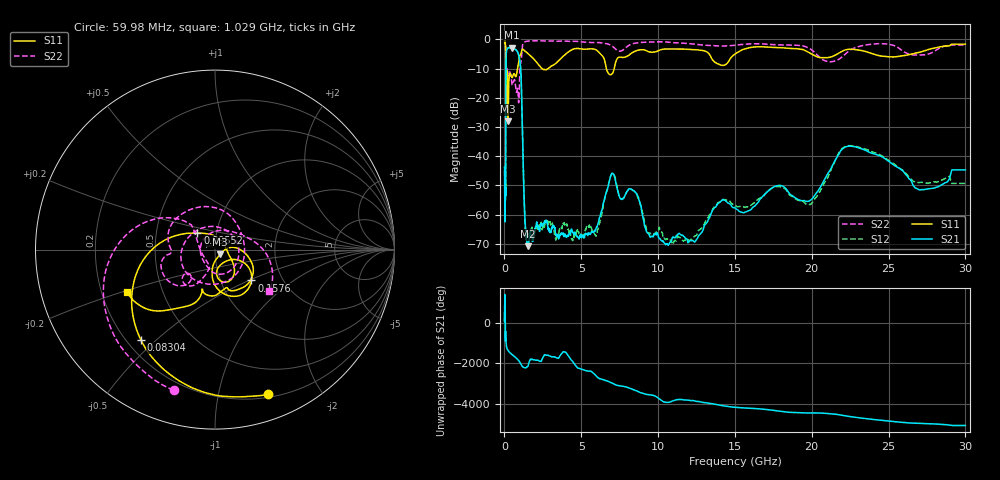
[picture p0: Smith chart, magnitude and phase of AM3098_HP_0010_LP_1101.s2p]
! Date/Time: Thu, Feb 28, 2019 8:33 AM
! Network Analyzer: Agilent Technologies E8364B Rev: A.07.50.67
! Sweep from 0.010 to 30.000 GHz, 1601 Points, Sweep Type: LOG
! Power Supply: 5.022 V, 0.002 A
# Hz S DB R 50
!freq MagS11 AngS11 MagS21 AngS21 MagS12 AngS12 MagS22 AngS22
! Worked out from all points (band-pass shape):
!   1601 points, 10 MHz to 30 GHz, reference 50 ohm
!   highest |S21| = -2.78 dB at 493.1 MHz (marker M1); lowest = -70.8 dB at 1.551 GHz (marker M2)
!   |S21| within 3 dB of the highest: 107.4 MHz to 945 MHz (837.6 MHz wide, 159 % of centre)
!   lowest |S11| = -28.1 dB at 232.8 MHz (marker M3), VSWR 1.08, Z = 52.9 - j2.81 ohm
!   |S11| at or under -10 dB: 92.13 MHz to 849.3 MHz (757.2 MHz wide, 161 % of centre); 2.455 GHz to 2.837 GHz (381.9 MHz wide, 14.4 % of centre); 6.636 GHz to 7.142 GHz (506.5 MHz wide, 7.35 % of centre)
!   |S22| runs from -22.7 to -0.4 dB; largest |S21 - S12| = 0.0097
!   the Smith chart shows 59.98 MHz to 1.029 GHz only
!   S11 on the Smith chart (normalised r, x): 59.98 MHz: 0.23, -1.41; 83.04 MHz: 0.26, -0.45; 95.52 MHz: 0.81, +0.15; 157.6 MHz: 1.40, -0.52; 1.029 GHz: 0.31, -0.21
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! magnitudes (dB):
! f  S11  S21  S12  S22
! 10 MHz  -0.3  -43.7  -45.1  -0.6
! 38.04 MHz  -0.5  -59.9  -57.4  -1.0
! 59.98 MHz  -1.3  -55.0  -50.7  -1.8
! 72.91 MHz  -2.0  -53.7  -51.5  -2.5
! 83.04 MHz  -3.7  -35.0  -34.3  -4.1
! 95.52 MHz  -17.4  -11.6  -11.6  -21.0
! 144.7 MHz  -15.0  -3.5  -3.5  -12.9
! 157.6 MHz  -11.5  -3.4  -3.4  -10.9
! 232.8 MHz  -28.1  -2.9  -2.9  -12.1
! 493.1 MHz  -13.1  -2.8  -2.8  -15.5
! 550.5 MHz  -12.4  -3.0  -3.0  -14.9
! 926.3 MHz  -7.8  -5.4  -5.3  -21.7
! 1.029 GHz  -5.3  -8.6  -8.6  -8.4
! 1.348 GHz  -4.0  -62.9  -64.8  -0.8
! 1.551 GHz  -4.9  -70.8  -66.5  -0.5
! 2.084 GHz  -7.7  -62.9  -65.1  -0.4
! 5.002 GHz  -3.3  -68.0  -66.8  -0.8
! 7.926 GHz  -5.9  -52.6  -52.6  -2.7
! 12.19 GHz  -3.5  -69.0  -68.2  -1.5
! 19.8 GHz  -4.4  -55.5  -56.5  -2.9
! 22.67 GHz  -3.4  -36.6  -36.5  -3.2
! 30 GHz  -1.6  -44.7  -49.3  -1.9
